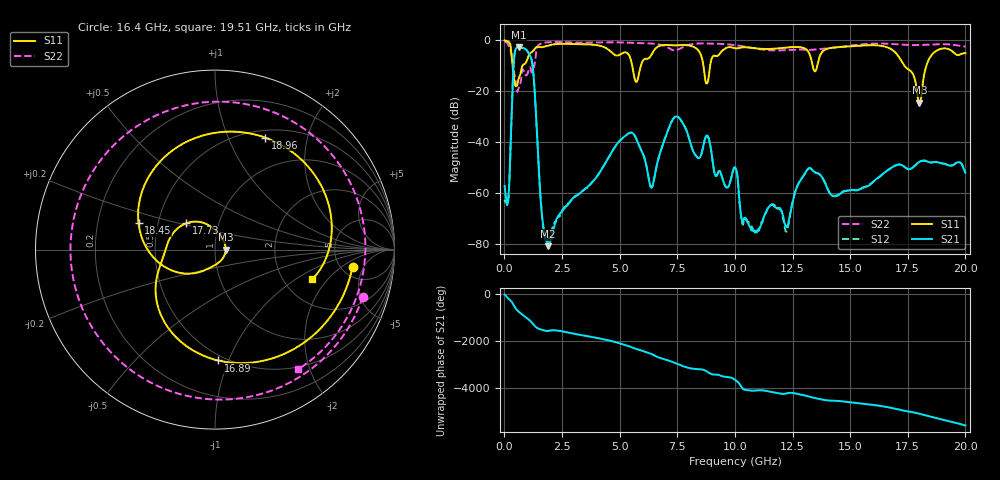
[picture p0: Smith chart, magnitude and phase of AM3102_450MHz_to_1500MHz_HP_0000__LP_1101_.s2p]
!Agilent Technologies,E8364B,MY43040894,A.07.50.67
!Agilent E8364B: A.07.50.67
!Date: Thursday, January 11, 2018 05:18:21
!Correction: S11(Full 2 Port(1,2))
!S21(Full 2 Port(1,2))
!S12(Full 2 Port(1,2))
!S22(Full 2 Port(1,2))
!S2P File: Measurements: S11, S21, S12, S22:
# Hz S  dB  R 50
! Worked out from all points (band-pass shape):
!   1601 points, 10 MHz to 20 GHz, reference 50 ohm
!   highest |S21| = -2.64 dB at 622.2 MHz (marker M1); lowest = -80.8 dB at 1.884 GHz (marker M2)
!   |S21| within 3 dB of the highest: 438.3 MHz to 1.088 GHz (650.2 MHz wide, 85.2 % of centre)
!   lowest |S11| = -24.4 dB at 18 GHz (marker M3), VSWR 1.13, Z = 56.4 - j0.0147 ohm
!   |S11| at or under -10 dB: 357.6 MHz to 780 MHz (422.5 MHz wide, 74.3 % of centre); 5.547 GHz to 5.92 GHz (372.3 MHz wide, 6.49 % of centre); 17.35 GHz to 18.31 GHz (951.6 MHz wide, 5.34 % of centre)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
!   |S22| runs from -20.2 to -0.5 dB; largest |S21 - S12| = 0.0051
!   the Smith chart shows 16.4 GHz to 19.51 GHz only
!   S11 on the Smith chart (normalised r, x): 16.4 GHz: 6.27, -3.05; 16.89 GHz: 0.46, -0.92; 17.73 GHz: 0.70, +0.21; 18.45 GHz: 0.39, +0.14; 18.96 GHz: 0.59, +1.38; 19.51 GHz: 2.86, -1.40
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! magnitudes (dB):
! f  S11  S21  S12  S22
! 10 MHz  -0.1  -57.1  -62.6  -0.5
! 159.9 MHz  -0.5  -63.2  -63.2  -1.6
! 622.2 MHz  -15.0  -2.6  -2.6  -18.7
! 1.197 GHz  -4.6  -8.4  -8.4  -12.5
! 1.622 GHz  -2.7  -68.0  -67.3  -1.2
! 1.884 GHz  -2.1  -80.8  -78.6  -0.8
! 3.346 GHz  -1.5  -59.5  -59.4  -0.9
! 5.407 GHz  -5.8  -36.4  -36.4  -0.9
! 6.682 GHz  -2.4  -46.4  -46.4  -1.5
! 7.481 GHz  -2.0  -29.9  -29.9  -3.8
! 10.01 GHz  -3.1  -49.9  -49.8  -1.9
! 10.9 GHz  -3.2  -74.9  -75.1  -3.2
! 13.34 GHz  -8.6  -50.7  -50.7  -3.7
! 16.4 GHz  -2.2  -52.6  -52.6  -1.3
! 16.68 GHz  -3.0  -50.7  -50.6  -1.4
! 16.89 GHz  -4.2  -49.4  -49.4  -1.5
! 17.73 GHz  -13.3  -49.9  -49.9  -1.9
! 18 GHz  -24.4  -47.7  -47.7  -1.9
! 18.45 GHz  -6.9  -47.8  -47.8  -1.7
! 18.96 GHz  -3.3  -48.2  -48.3  -1.5
! 19.51 GHz  -4.9  -48.7  -48.7  -1.8
! 20 GHz  -5.0  -51.9  -52.0  -2.4
